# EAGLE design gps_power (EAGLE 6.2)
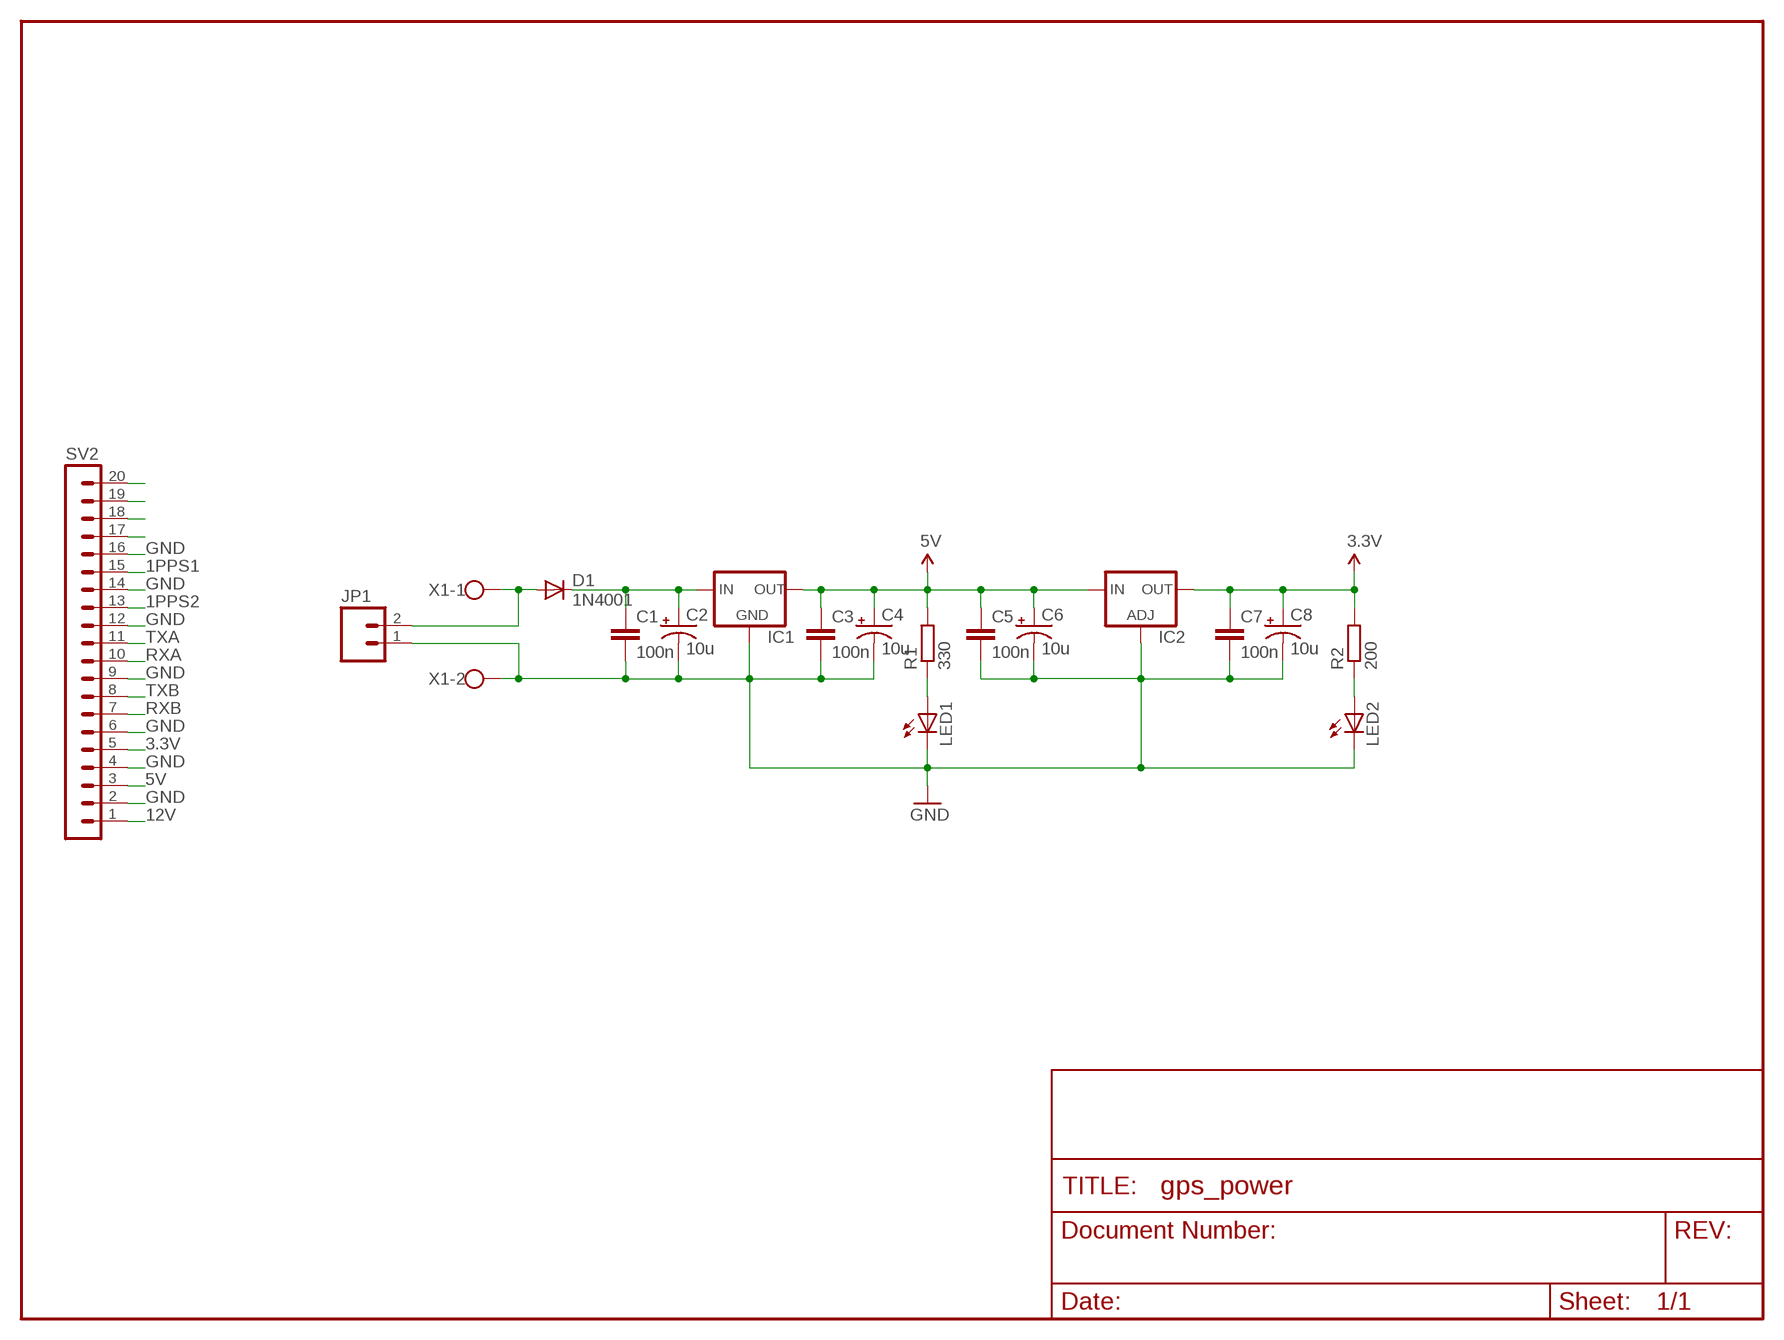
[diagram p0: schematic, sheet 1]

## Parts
C1  100n  CAPPTH1  [CAP-PTH-5MM]
C2  10u  CAP_POLPTH2  [CPOL-RADIAL-10UF-25V]
C3  100n  CAPPTH1  [CAP-PTH-5MM]
C4  10u  CAP_POLPTH2  [CPOL-RADIAL-10UF-25V]
C5  100n  CAPPTH1  [CAP-PTH-5MM]
C6  10u  CAP_POLPTH2  [CPOL-RADIAL-10UF-25V]
C7  100n  CAPPTH1  [CAP-PTH-5MM]
C8  10u  CAP_POLPTH2  [CPOL-RADIAL-10UF-25V]
D1  1N4001  DIODEPTH  [DIODE-1N4001]
IC1  78MXXS  [78MXXS]
IC2  LM317TS  [317TS]
JP1  M02PTH3  [1X02_LONGPADS]
LED1  LED5MM  [LED5MM]
LED2  LED5MM  [LED5MM]
R1  330  R-EU_0204/7  [0204/7]
R2  200  R-EU_0204/7  [0204/7]
SV2  MA20-1W  [MA20-1W]
X1  W237-102  [W237-102]

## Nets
1PPS1: SV2.15
1PPS2: SV2.13
3.3V: C7.1 C8.1(+) IC2.2(OUT) R2.2 SV2.5
5V: C3.1 C4.1(+) C5.1 C6.1(+) IC1.OUT IC2.3(IN) R1.2 SV2.3
12V: SV2.1
GND: C1.2 C2.2(-) C3.2 C4.2(-) C5.2 C6.2(-) C7.2 C8.2(-) IC1.GND IC2.1(ADJ) JP1.1 LED1.K(C) LED2.K(C) SV2.2 SV2.4 SV2.6 SV2.9 SV2.12 SV2.14 SV2.16 X1.2
N$1: D1.A JP1.2 X1.1
N$2: C1.1 C2.1(+) D1.C IC1.IN
N$4: LED1.A R1.1
N$6: LED2.A R2.1
N$17: SV2.17
N$18: SV2.18
N$19: SV2.19
N$20: SV2.20
RXA: SV2.10
RXB: SV2.7
TXA: SV2.11
TXB: SV2.8

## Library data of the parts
C1 C3 C5 C7 = SparkFun:CAP: Capacitor
C2 C4 C6 C8 = SparkFun:CAP_POL: Capacitor Polarized
D1 = SparkFun:DIODE: Diode
IC1 = v-reg:78MXXS: VOLTAGE REGULATOR
IC2 = v-reg:LM317TS: VOLTAGE REGULATOR
JP1 = SparkFun:M02: Header 2
LED1 LED2 = SparkFun:LED: LEDs
R1 R2 = resistor:R-EU_: RESISTOR, European symbol
SV2 = con-lstb:MA20-1W: PIN HEADER; OC_FARNELL: unknown; OC_NEWARK: unknown
X1 = con-wago-500:W237-102: WAGO SCREW CLAMP; MPN: 237-102; OC_FARNELL: unknown; OC_NEWARK: 70K9898

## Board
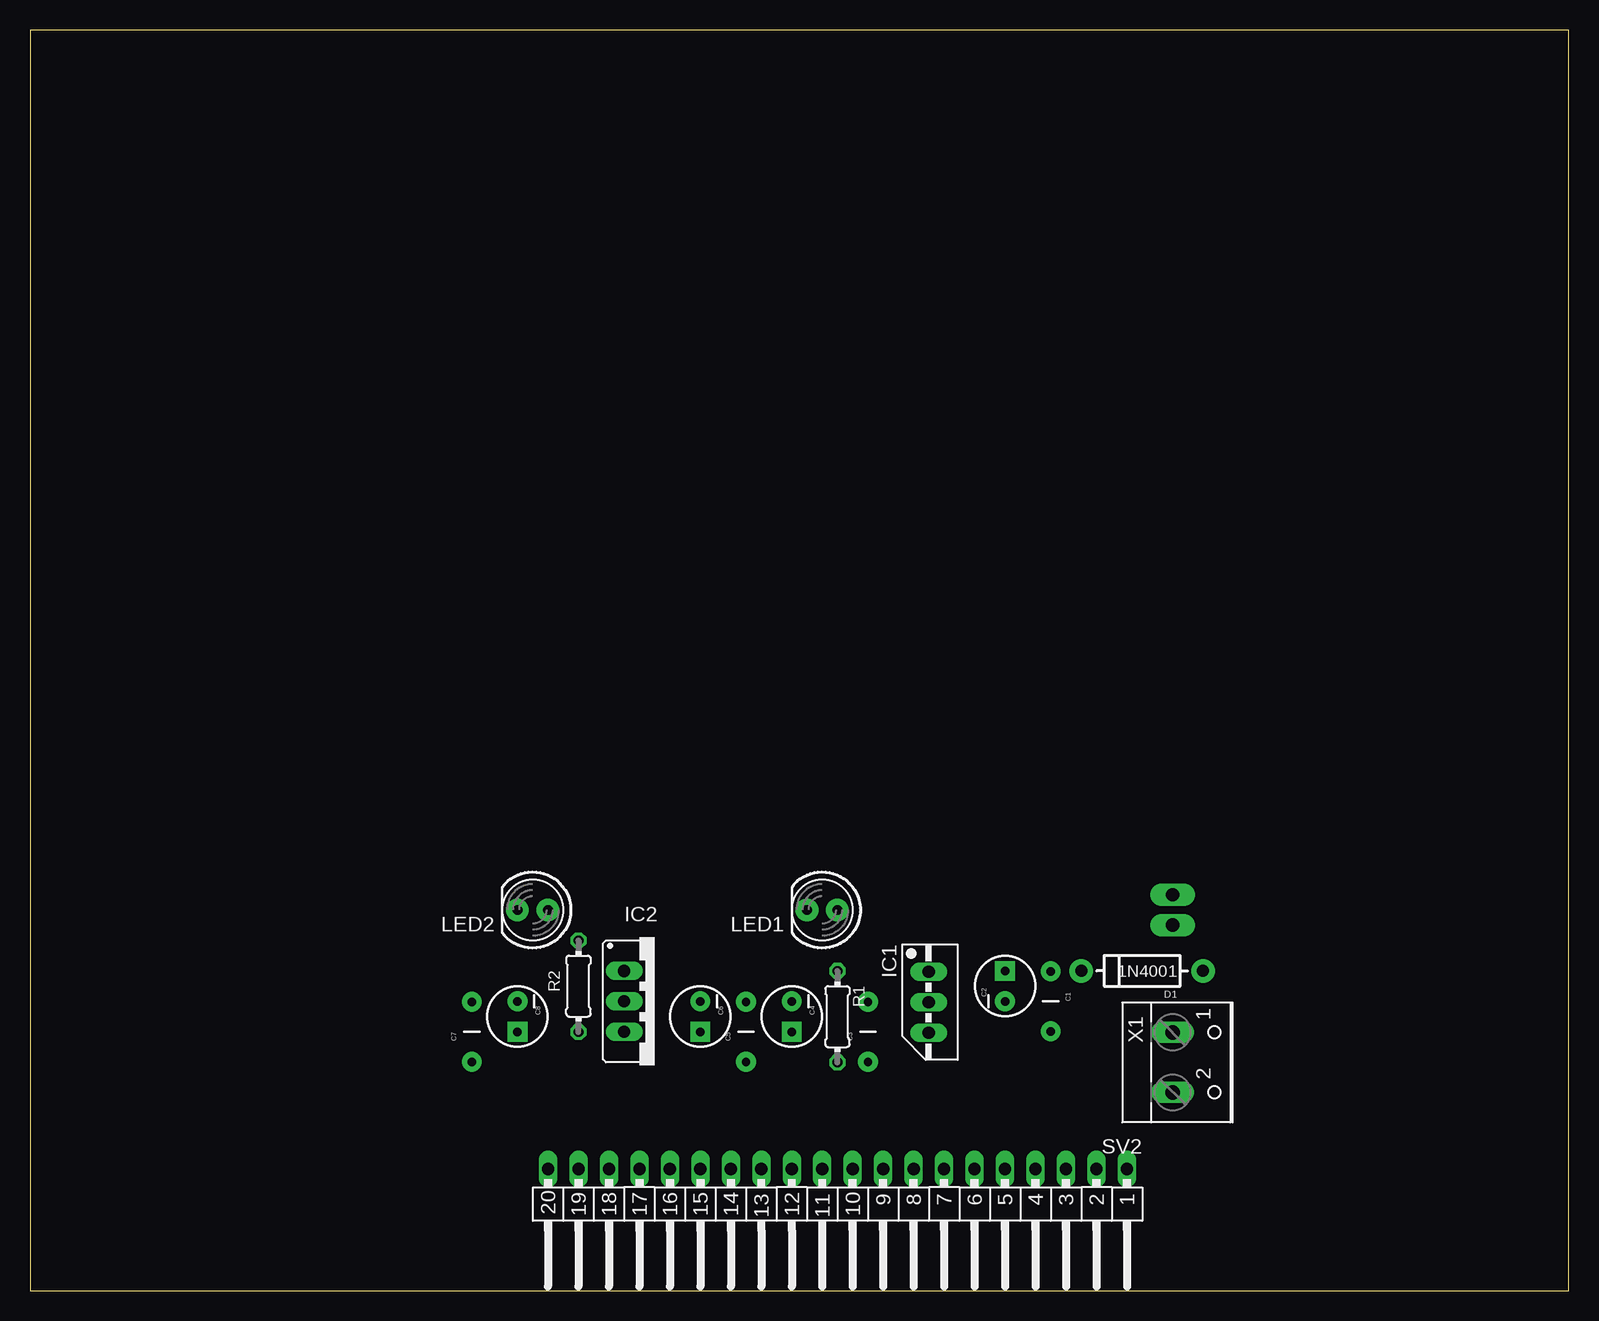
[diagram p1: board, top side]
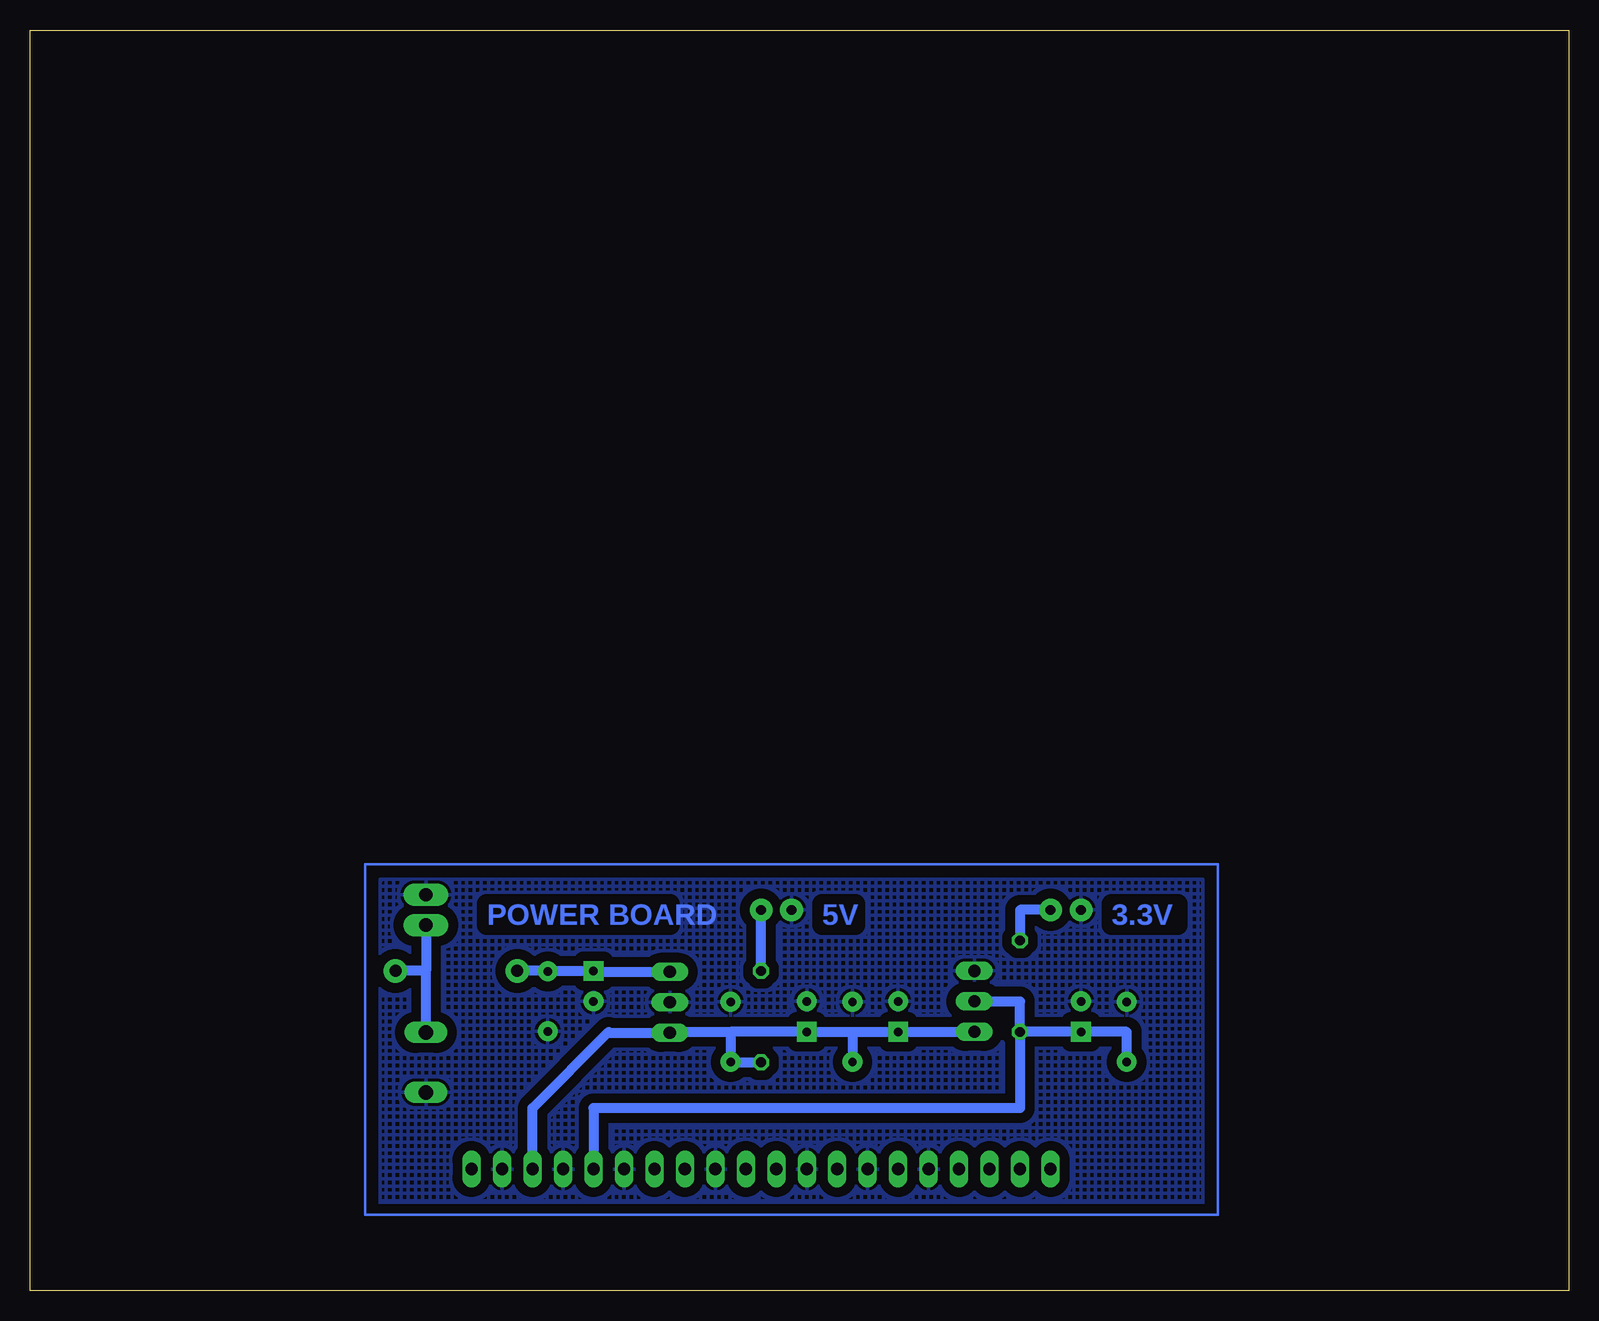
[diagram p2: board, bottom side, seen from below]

Size 128.25 x 105.08 mm. Coordinates in mm from the lower left corner, seen from the top.
Outline: 0,0 128.25,0 128.25,105.08 0,105.08 0,0
Copper layers (1*16): Top 0.035mm / dielectric 1.5mm / Bottom 0.035mm
Design rules: minimum track width 10mil, minimum drill 24mil, track to track 8mil, track to pad 8mil, pad to pad 8mil, via to via 8mil, smd to smd 8mil, copper to edge 40mil, drill to drill 8mil, minimum pad ring 10mil, minimum via ring 8mil, stop-mask expansion 4mil, vias tented up to drill 0mil, thermal gap 10mil

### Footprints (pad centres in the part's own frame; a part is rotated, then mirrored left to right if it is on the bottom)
CAP-PTH-5MM = drill 0.7 pad 1.651: 1 -2.5,0; 2 2.5,0
CPOL-RADIAL-10UF-25V = drill 0.7 pad 1.651 square: 1 1.27,0 | drill 0.7 pad 1.651: 2 -1.27,0
DIODE-1N4001 = drill 1 pad 1.981: A -5.08,0; C 5.08,0
78MXXS = drill 1.016 long: GND 0,-2.54; IN -2.54,-2.54; OUT 2.54,-2.54
317TS = drill 1.016 long: 1 -2.54,-2.54; 2 0,-2.54; 3 2.54,-2.54
1X02_LONGPADS = drill 1.118 pad 1.88 long: 1 0,0; 2 2.54,0
LED5MM = drill 0.813 pad 1.88: A -1.27,0; K 1.27,0
0204/7 = drill 0.813 octagon: 1 -3.81,0; 2 3.81,0
MA20-1W = drill 1.016 long: 1 -24.13,0; 2 -21.59,0; 3 -19.05,0; 4 -16.51,0; 5 -13.97,0; 6 -11.43,0; 7 -8.89,0; 8 -6.35,0; 9 -3.81,0; 10 -1.27,0; 11 1.27,0; 12 3.81,0; 13 6.35,0; 14 8.89,0; 15 11.43,0; 16 13.97,0; 17 16.51,0; 18 19.05,0; 19 21.59,0; 20 24.13,0
W237-102 = drill 1.194 long: 1 -2.5,-1.27; 2 2.5,-1.27

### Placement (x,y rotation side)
C1  85.09,24.13 270 top
C2  81.28,25.4 90 top
C3  69.85,21.59 90 top
C4  63.5,22.86 270 top
C5  59.69,21.59 90 top
C6  55.88,22.86 270 top
C7  36.83,21.59 90 top
C8  40.64,22.86 270 top
D1  92.71,26.67 180 top
IC1  77.45,24.05 270 top
IC2  52.07,24.13 270 top
JP1  95.25,33.02 270 top
LED1  66.04,31.75 180 top
LED2  41.91,31.75 180 top
R1  67.31,22.86 270 top
R2  45.72,25.4 270 top
SV2  67.31,10.16 180 top
X1  96.52,19.05 270 top

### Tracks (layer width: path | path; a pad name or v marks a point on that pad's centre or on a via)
3.3V
  Bottom 0.813: C7.1 36.83,21.59 C8.1 R2.2 | R2.2 45.72,24.13 IC2.2 | R2.2 45.72,15.24 81.28,15.24 SV2.5
5V
  Bottom 0.813: 69.85,21.59 74.83,21.59 IC1.OUT 79.93,21.51 80.01,21.59 86.36,15.24 SV2.3 | 69.85,21.59 C3.1 | C3.1 69.85,19.05 | C3.1 69.81,19.05 R1.2 | 69.85,21.59 C4.1 59.69,21.59 | 59.69,21.59 C5.1 | 59.69,21.59 C6.1 IC2.3
GND
  pour Bottom (isolate 0.813, rank 2, hatched): 30.48,34.29 99.06,34.29 99.06,6.35 30.48,6.35
N$1
  Bottom 0.813: X1.1 95.25,26.67 | 95.25,26.67 D1.A | JP1.2 95.25,26.67
N$2
  Bottom 0.813: D1.C 85.13,26.67 C1.1 85.05,26.67 C2.1 81.2,26.59 IC1.IN
N$4
  Bottom 0.813: R1.1 LED1.A
N$5
  Bottom 0.2: 100.33,6.35 29.21,6.35 29.21,35.56 100.33,35.56 100.33,6.35
N$6
  Bottom 0.813: LED2.A 45.72,31.75 R2.1

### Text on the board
Bottom: 3.3V | 5V | POWER BOARD
_tNames: LED2 | IC2 | LED1 | IC1 | R2 | R1 | C1 | D1 | C8 | C6 | C4 | C2 | X1 | C7 | C5 | C3 | SV2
